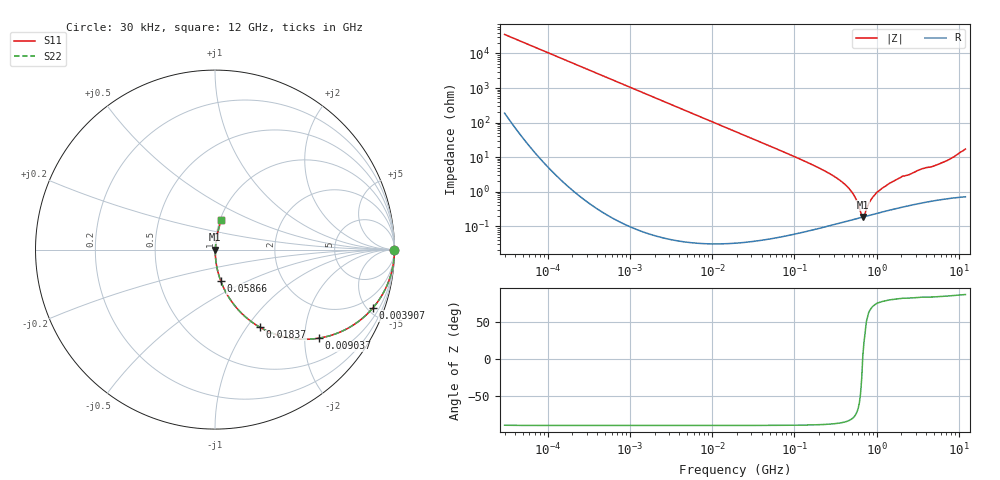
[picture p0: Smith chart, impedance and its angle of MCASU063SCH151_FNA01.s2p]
! MCASU063SCH151_FNA01  S-PARAMETER MODEL  ( General Type )
! Model Generated by TAIYO YUDEN Corporation (http://www.ty-top.com)
! Version 1.0
! TAIYO YUDEN Control No. 181120
! Copyright(c) 2018 TAIYO YUDEN CO.,LTD. All Rights Reserved.
! Product Description (link to TY-COMPAS)
! https://ds.yuden.co.jp/TYCOMPAS/or/detail?pn=MCASU063SCH151JFNA01&u=M
! Products Name : Multilayer Ceramic Capacitors
! Characteristics :
!  Capacitance : 150 pF , Rated Voltage : 50V , TCC : CH / C0H
!  Case Size : 0.6 x 0.3 / 0.024 x 0.012 [mm/inch] , Thickness : 0.3 / 0.012 [mm/inch]
!  (Conditions: Temperature = 25 degC , DC Bias Current/Voltage = 0A / 0V)
! External Node Assignments :
!  1  o---| |---o  2
! GND o---------o GND
! Frequency Range : 0.03MHz  -  12000MHz  [ 401 STEP ]
# MHz S RI R 50
! Freq[MHz].  S11 Real  S11 Imag  S21 Real  S21 Imag  S12 Real  S12 Imag  S22 Real  S22 Imag
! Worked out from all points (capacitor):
!   401 points, 30 kHz to 12 GHz, reference 50 ohm
!   read as one part in series: C = 150 pF near 32 kHz
!   lowest |Z| = 186 mohm at 680.3 MHz (marker M1)
!   series resonance near 676.7 MHz, so ESL is about 370 pH
!   S11 on the Smith chart (normalised r, x): 30 kHz: open; 3.907 MHz: 1.00, -5.43; 9.037 MHz: 1.00, -2.35; 18.37 MHz: 1.00, -1.15; 58.66 MHz: 1.00, -0.36; 12 GHz: 1.01, +0.34
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0.03  1 -0.00283  2.3e-05 0.00283  2.3e-05 0.00283  1 -0.00283
0.260295  0.9994 -0.0245  0.000605 0.0245  0.000605 0.0245  0.9994 -0.0245
2.258455  0.9566 -0.2036  0.0434 0.2036  0.0434 0.2036  0.9566 -0.2036
3.907499  0.8805 -0.3243  0.1195 0.3243  0.1195 0.3243  0.8805 -0.3243
9.037177  0.5795 -0.4935  0.4205 0.4935  0.4205 0.4935  0.5795 -0.4935
18.37156  0.25 -0.4327  0.75 0.4327  0.75 0.4327  0.25 -0.4327
18.97367  0.2381 -0.4256  0.7619 0.4256  0.7619 0.4256  0.2381 -0.4256
31.78584  0.1001 -0.2996  0.8999 0.2996  0.8999 0.2996  0.1001 -0.2996
58.65857  0.0316 -0.1738  0.9684 0.1738  0.9684 0.1738  0.0316 -0.1738
164.6252  0.00443 -0.0603  0.9956 0.0603  0.9956 0.0603  0.00443 -0.0603
294.1636  0.00195 -0.0292  0.9981 0.0292  0.9981 0.0292  0.00195 -0.0292
433.1624  0.0016 -0.0144  0.9984 0.0144  0.9984 0.0144  0.0016 -0.0144
542.8588  0.00166 -0.00697  0.9983 0.00697  0.9983 0.00697  0.00166 -0.00697
637.8412  0.00178 -0.00188  0.9982 0.00188  0.9982 0.00188  0.00178 -0.00188
680.3351  0.00185 0.000179  0.9981 -0.000179  0.9981 -0.000179  0.00185 0.000179
725.66  0.00193 0.00141  0.9981 -0.00141  0.9981 -0.00141  0.00193 0.00141
825.5698  0.00211 0.00471  0.9979 -0.00471  0.9979 -0.00471  0.00211 0.00471
939.2353  0.00232 0.00749  0.9977 -0.00749  0.9977 -0.00749  0.00232 0.00749
1428.372  0.00319 0.017  0.9968 -0.017  0.9968 -0.017  0.00319 0.017
3303.507  0.00631 0.042  0.9937 -0.042  0.9937 -0.042  0.00631 0.042
6935.754  0.0118 0.0749  0.9882 -0.0749  0.9882 -0.0749  0.0118 0.0749
12000  0.035 0.1642  0.965 -0.1642  0.965 -0.1642  0.035 0.1642
